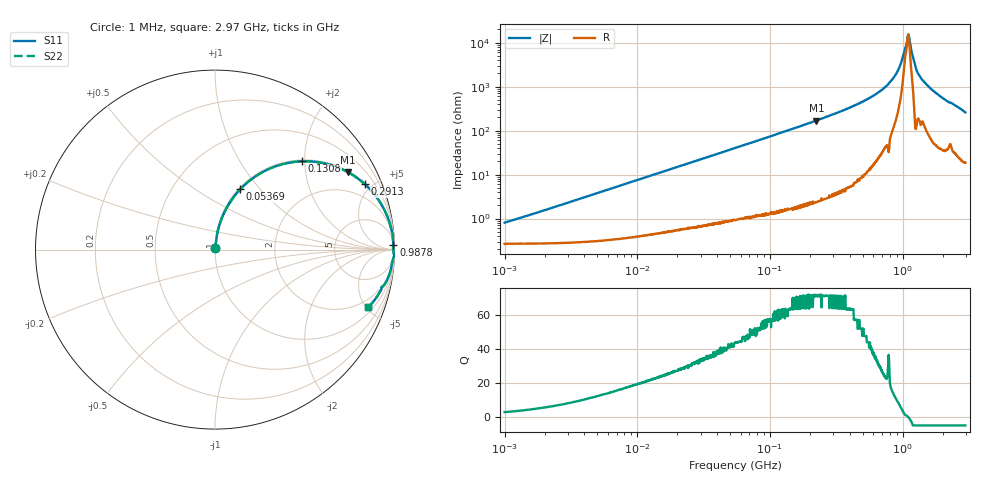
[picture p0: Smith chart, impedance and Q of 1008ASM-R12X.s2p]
!s-Parameter Generated by FASTRON Sdn. Bhd.
!FASTRON P/N : 1008ASM-R12X
!Keysight Technologies: E4991B_MY54100416_A.01.15
!Date: Mon Nov 20 16:05:34 2023
!Version  :Rev00  Wed Nov 22 15:12:09 2023
!Data & Calibration Information:
!Freq  S11  S21  S12  S22
!PortZ  Port1:50+j0  Port2:50+j0
!When reading reference impedance value at option line is always used.
! Remarks : This data is being provided solely for informational purposes.
# Hz S dB R 50
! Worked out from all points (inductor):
!   1599 points, 1 MHz to 2.97 GHz, reference 50 ohm
!   read as one part in series: L = 122 nH near 1.051 MHz
!   highest Q = 71.9 at 223.5 MHz (marker M1), where L = 121 nH
!   self-resonance near 1.097 GHz
!   S11 on the Smith chart (normalised r, x): 1 MHz: 1.01, +0.02; 53.69 MHz: 1.02, +0.79; 130.8 MHz: 1.03, +1.94; 291.3 MHz: 1.06, +4.55; 987.8 MHz: 19, +79; 2.97 GHz: 1.37, -5.21
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1000000  -41.90 70.4  -0.02 -0.4  -0.02 -0.4  -41.90 70.4
3804036  -30.80 82.6  -0.03 -1.6  -0.03 -1.6  -30.80 82.6
1.439846e7  -19.40 81.4  -0.09 -6.1  -0.09 -6.1  -19.40 81.4
5.368684e7  -8.75 67.3  -0.70 -21.4  -0.70 -21.4  -8.75 67.3
5.477226e7  -8.60 66.9  -0.72 -21.8  -0.72 -21.8  -8.60 66.9
1.308271e8  -3.22 45.5  -2.94 -43.6  -2.94 -43.6  -3.22 45.5
2.073156e8  -1.54 32.4  -5.43 -56.8  -5.43 -56.8  -1.54 32.4
2.234756e8  -1.35 30.3  -5.94 -58.9  -5.94 -58.9  -1.35 30.3
2.913464e8  -0.81 23.6  -7.96 -65.6  -7.96 -65.6  -0.81 23.6
5.258324e8  -0.21 11.4  -14.10 -77.4  -14.10 -77.4  -0.21 11.4
6.652545e8  -0.11 7.4  -17.80 -80.7  -17.80 -80.7  -0.11 7.4
7.846996e8  -0.05 4.8  -21.50 -83.6  -21.50 -83.6  -0.05 4.8
9.0272e8  -0.05 2.7  -26.40 -81.5  -26.40 -81.5  -0.05 2.7
9.878038e8  -0.05 1.4  -32.20 -75.8  -32.20 -75.8  -0.05 1.4
1.075512e9  -0.07 0.3  -40.40 -34.8  -40.40 -34.8  -0.07 0.3
1.108292e9  -0.05 -0.1  -43.70 16.0  -43.70 16.0  -0.05 -0.1
1.130699e9  -0.05 -0.4  -40.90 50.2  -40.90 50.2  -0.05 -0.4
1.194682e9  -0.04 -1.2  -33.50 77.9  -33.50 77.9  -0.04 -1.2
1.262285e9  -0.02 -2.3  -28.10 85.1  -28.10 85.1  -0.02 -2.3
1.409185e9  -0.09 -4.0  -23.10 79.4  -23.10 79.4  -0.09 -4.0
1.970482e9  -0.23 -9.8  -15.40 76.5  -15.40 76.5  -0.23 -9.8
2.970126e9  -0.80 -20.4  -9.11 65.5  -9.11 65.5  -0.80 -20.4
